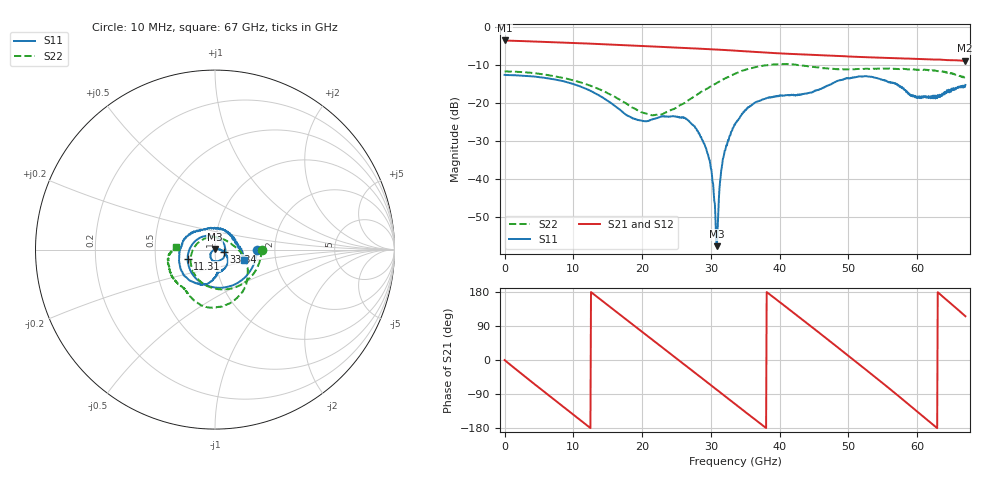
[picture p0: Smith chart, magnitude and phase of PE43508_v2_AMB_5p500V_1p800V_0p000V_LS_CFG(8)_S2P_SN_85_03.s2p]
!Keysight Technologies,N5227A,US51270237,A.10.43.00
!Date: Wednesday, August 22, 2018 17:07:21
!Correction: S11(Full 2 Port(1,3))
!S31(Full 2 Port(1,3))
!S13(Full 2 Port(1,3))
!S33(Full 2 Port(1,3))
!S2P File: Measurements: S11, S31, S13, S33:
# Hz S  dB  R 50
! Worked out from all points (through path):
!   801 points, 10 MHz to 67 GHz, reference 50 ohm
!   highest |S21| = -3.59 dB at 10 MHz (marker M1); lowest = -8.9 dB at 66.92 GHz (marker M2)
!   group delay of S21, straight-line fit = 39.5 ps
!   lowest |S11| = -57.7 dB at 30.83 GHz (marker M3), VSWR 1.00, Z = 49.9 + j0.0813 ohm
!   |S11| at or under -10 dB: start of sweep to end of sweep
!   |S22| runs from -23.3 to -9.8 dB; largest |S21 - S12| = 0.003
!   S11 on the Smith chart (normalised r, x): 10 MHz: 1.61, -0.01; 11.31 GHz: 0.73, -0.08; 33.34 GHz: 1.10, -0.02; 67 GHz: 1.38, -0.16
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1e7  -12.64 -0.4  -3.59 -0.2  -3.59 -0.2  -11.71 -0.3
5.70415e9  -13.38 -83.9  -3.95 -83.1  -3.94 -83.0  -12.51 -65.0
8.216275e9  -14.17 -119.1  -4.13 -119.0  -4.12 -118.9  -13.34 -92.6
1.123082e10  -15.83 -160.5  -4.34 -161.8  -4.33 -161.8  -14.70 -125.2
1.131456e10  -15.89 -161.7  -4.34 -163.0  -4.34 -163.0  -14.75 -126.2
1.40779e10  -18.39 156.9  -4.55 157.9  -4.54 157.9  -16.65 -157.7
1.734366e10  -22.68 94.5  -4.82 111.8  -4.81 111.8  -19.79 158.9
2.236791e10  -23.86 -36.1  -5.25 41.0  -5.25 41.1  -23.12 67.5
2.521499e10  -23.76 -87.7  -5.49 1.0  -5.48 1.1  -20.93 25.6
2.822954e10  -28.03 -128.7  -5.74 -41.4  -5.74 -41.3  -17.56 -1.1
2.982055e10  -35.08 -150.3  -5.88 -63.9  -5.87 -63.8  -15.84 -12.8
3.08254e10  -57.66 141.6  -5.98 -78.1  -5.98 -78.0  -14.80 -20.2
3.183025e10  -34.29 3.5  -6.08 -92.3  -6.07 -92.2  -13.78 -28.4
3.333752e10  -26.20 -12.9  -6.24 -113.6  -6.23 -113.6  -12.48 -40.2
3.3505e10  -25.72 -15.9  -6.26 -116.0  -6.25 -116.0  -12.34 -41.5
3.861299e10  -18.61 -63.6  -6.84 172.3  -6.84 172.3  -10.00 -80.8
4.472582e10  -17.21 -86.4  -7.36 86.3  -7.35 86.4  -10.52 -116.7
5.033624e10  -13.42 -117.0  -7.83 6.1  -7.83 6.1  -11.14 -130.6
5.586291e10  -14.61 174.1  -8.18 -74.1  -8.18 -74.4  -10.97 -147.5
6.180828e10  -18.41 53.3  -8.56 -163.3  -8.59 -163.4  -11.45 -167.2
6.691626e10  -15.87 -18.0  -8.93 116.9  -8.98 117.0  -13.20 177.7
6.7e10  -15.28 -18.9  -8.92 115.5  -8.97 115.7  -13.30 176.6
